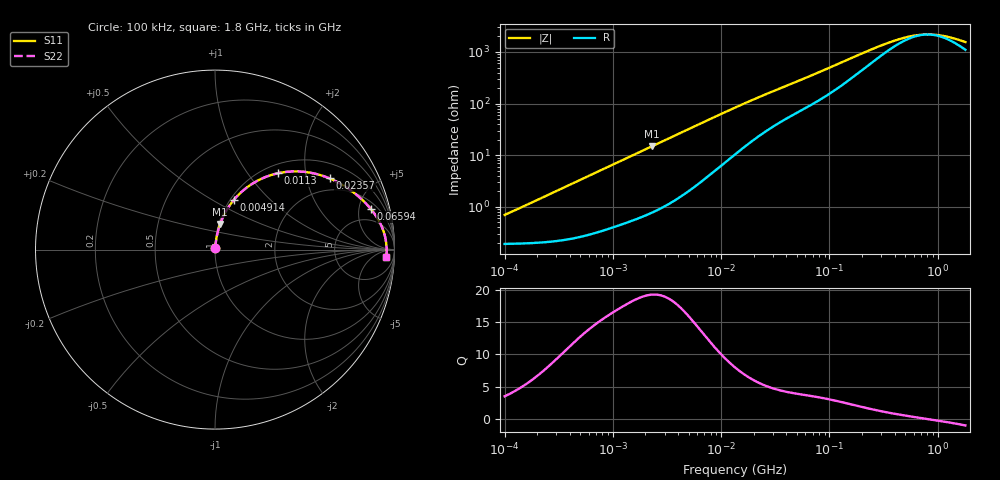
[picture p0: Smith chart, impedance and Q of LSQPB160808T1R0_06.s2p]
! LSQPB160808T1R0_06  S-PARAMETER MODEL  ( General Type )
! Model Generated by TAIYO YUDEN Corporation (http://www.ty-top.com)
! Version 1.0
! TAIYO YUDEN Control No. 110726NG25SE-FKC
! Copyright(c) 2011 TAIYO YUDEN CO.,LTD. All Rights Reserved.
! Product Description (link to TY-COMPAS)
! https://ds.yuden.co.jp/TYCOMPAS/or/detail?pn=LSQPB160808T1R0M06&u=M
! Products Name : Inductors
! Characteristics :
!  Inductance : 1.0 uH , SRF(min) : 550 MHz , DC Resistance(max) : 0.2444 Ohm
!  Rated Current : Saturation :890 mA , Temp Rise : 680 mA (40 degC)
!  Case Size : 1.6 x 0.8 / 0.063 x 0.031 [mm/inch] , Thickness : 0.8 / 0.031 [mm/inch]
!  (Conditions: Temperature = 25 degC , DC Bias Current/Voltage = 0A / 0V)
! External Node Assignments :
!  1  o---GGG---o  2
! GND o---------o GND
! Frequency Range : 0.1MHz  -  1800MHz  [ 402 STEP ]
# MHz S RI R 50
! Freq[MHz].  S11 Real  S11 Imag  S21 Real  S21 Imag  S12 Real  S12 Imag  S22 Real  S22 Imag
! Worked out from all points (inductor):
!   401 points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, 100 kHz to 1.8 GHz, reference 50 ohm
!   read as one part in series: L = 1.07 uH near 105 kHz
!   highest Q = 19.2 at 2.3 MHz (marker M1), where L = 1.03 uH
!   self-resonance near 802.3 MHz
!   S11 on the Smith chart (normalised r, x): 100 kHz: 1.00, +0.01; 4.914 MHz: 1.04, +0.63; 11.3 MHz: 1.16, +1.41; 23.57 MHz: 1.51, +2.75; 65.94 MHz: 2.83, +6.57; 1.8 GHz: 23, -22
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0.1  0.00196 0.00669  0.998 -0.00669  0.998 -0.00669  0.00196 0.00669
0.147983  0.00205 0.0099  0.998 -0.0099  0.998 -0.0099  0.00205 0.0099
0.516129  0.00382 0.0342  0.9962 -0.0342  0.9962 -0.0342  0.00382 0.0342
1.187015  0.0104 0.0766  0.9896 -0.0766  0.9896 -0.0766  0.0104 0.0766
2.299785  0.0288 0.1433  0.9712 -0.1433  0.9712 -0.1433  0.0288 0.1433
2.66389  0.0368 0.1641  0.9632 -0.1641  0.9632 -0.1641  0.0368 0.1641
3.662795  0.0634 0.2176  0.9366 -0.2176  0.9366 -0.2176  0.0634 0.2176
4.914404  0.1045 0.2763  0.8955 -0.2763  0.8955 -0.2763  0.1045 0.2763
7.452807  0.2023 0.3635  0.7977 -0.3635  0.7977 -0.3635  0.2023 0.3635
11.30236  0.3508 0.4254  0.6492 -0.4254  0.6492 -0.4254  0.3508 0.4254
13.41641  0.4211 0.4351  0.5789 -0.4351  0.5789 -0.4351  0.4211 0.4351
17.56533  0.5311 0.4285  0.4689 -0.4285  0.4689 -0.4285  0.5311 0.4285
23.56755  0.6384 0.3968  0.3616 -0.3968  0.3616 -0.3968  0.6384 0.3968
38.46609  0.773 0.3178  0.227 -0.3178  0.227 -0.3178  0.773 0.3178
65.93531  0.8675 0.2272  0.1325 -0.2272  0.1325 -0.2272  0.8675 0.2272
69.24595  0.8739 0.2193  0.1261 -0.2193  0.1261 -0.2193  0.8739 0.2193
137.4876  0.9311 0.1232  0.0689 -0.1232  0.0689 -0.1232  0.9311 0.1232
357.3983  0.9533 0.0411  0.0467 -0.0411  0.0467 -0.0411  0.9533 0.0411
555.4434  0.9556 0.0173  0.0444 -0.0173  0.0444 -0.0173  0.9556 0.0173
802.0705  0.9562 1.41e-05  0.0438 -1.41e-05  0.0438 -1.41e-05  0.9562 1.41e-05
1158.204  0.9561 -0.0173  0.0439 0.0173  0.0439 0.0173  0.9561 -0.0173
1800  0.9547 -0.0414  0.0453 0.0414  0.0453 0.0414  0.9547 -0.0414
